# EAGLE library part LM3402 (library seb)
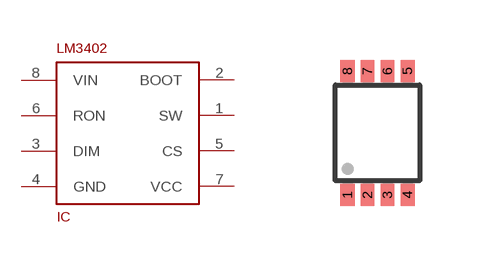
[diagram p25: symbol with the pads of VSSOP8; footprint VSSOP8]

Designator prefix IC

## LM3402  [VSSOP8]
1  SW
2  BOOT
3  DIM
4  GND
5  CS
6  RON
7  VCC
8  VIN

## Footprint VSSOP8 (pad centres in mm)
smd 0.35 x 0.55: 1 -0.75,-1.55; 2 -0.25,-1.55; 3 0.25,-1.55; 4 0.75,-1.55; 5 0.75,1.55; 6 0.25,1.55; 7 -0.25,1.55; 8 -0.75,1.55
